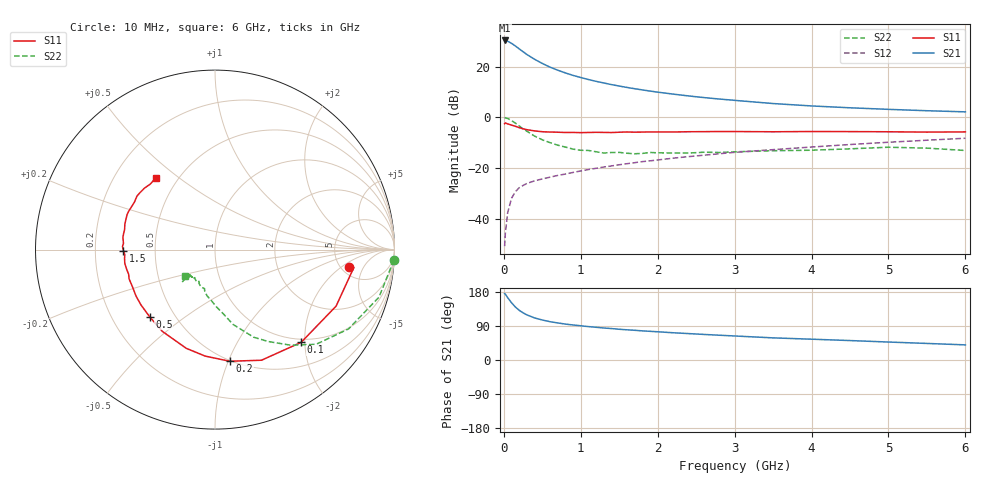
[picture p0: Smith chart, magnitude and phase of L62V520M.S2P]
!  INFINEON TECHNOLOGIES Small Signal Semiconductors
! BFR380L3 , Si-NPN RF-Transistor in TSLP-3-1
!  Vce=2.5 V,  Ic=20 mA
! Common Emitter S-Parameters:  07. March 2005
#  GHz  S  MA  R  50
! f  S11  S21  S12  S22
! GHz  Mag  Ang  Mag  Ang  Mag  Ang  Mag  Ang
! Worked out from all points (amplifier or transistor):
!   36 points, 10 MHz to 6 GHz, reference 50 ohm
!   highest |S21| = 30.3 dB at 10 MHz (marker M1)
!   |S21| within 3 dB of that: start of sweep to 185.8 MHz
!   unconditionally stable (mu >= 1): 1.909 GHz to 4.837 GHz
!   at 250 MHz: K = 0.37, MSG = 26.4 dB, |S12| = -26.8 dB
!   at 1.4 GHz: K = 0.95, MSG = 16.0 dB, |S12| = -19.1 dB
!   at 6 GHz: K = 0.97, MSG = 5.2 dB, |S12| = -8.2 dB
!   S11 on the Smith chart (normalised r, x): 10 MHz: 5.84, -2.59; 100 MHz: 0.94, -1.92; 200 MHz: 0.49, -1.01; 500 MHz: 0.36, -0.37; 1.5 GHz: 0.32, -0.00; 6 GHz: 0.38, +0.42
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0.01  0.7505 -7.4  32.83 175.0  0.0029 87.4  0.9974 -3.3
0.02  0.7797 -7.4  32.75 173.8  0.0053 84.4  0.981 -6.7
0.05  0.7446 -25.0  31.62 164.5  0.0133 81.4  0.9511 -16.2
0.1  0.7053 -47.1  28.82 151.1  0.0255 69.1  0.8655 -30.7
0.15  0.6686 -67.2  25.57 139.8  0.0344 62.0  0.772 -43.1
0.2  0.6274 -82.5  22.38 131.1  0.0411 58.7  0.6799 -51.6
0.25  0.5959 -95.3  19.7 124.5  0.0456 53.7  0.592 -59.9
0.3  0.5727 -106.3  17.35 119.0  0.0499 52.7  0.5335 -66.2
0.4  0.5419 -122.8  13.95 111.0  0.0563 50.6  0.4283 -76.5
0.5  0.522 -134.3  11.57 105.5  0.0613 50.9  0.3618 -82.5
0.6  0.5148 -143.3  9.787 101.1  0.0664 51.9  0.3182 -88.7
0.8  0.5044 -155.9  7.529 94.8  0.0765 54.3  0.2602 -100.0
0.9  0.5057 -161.3  6.72 92.4  0.0823 55.7  0.2372 -104.0
1.1  0.5046 -167.8  5.574 88.1  0.0939 57.8  0.2233 -110.0
1.5  0.5103 -179.4  4.15 81.1  0.1166 60.6  0.2045 -120.3
1.8  0.5139 174.3  3.483 76.9  0.1344 61.5  0.195 -125.8
2.2  0.516 167.4  2.878 71.9  0.1572 62.4  0.1992 -129.3
2.8  0.5272 158.2  2.303 65.4  0.1921 63.2  0.2037 -136.2
3.5  0.521 149.4  1.875 58.4  0.2316 61.9  0.2204 -135.7
4.5  0.5249 142.9  1.547 51.3  0.2921 61.0  0.2402 -135.6
5.5  0.5131 134.7  1.354 43.7  0.3552 57.7  0.248 -135.7
6  0.5182 129.3  1.286 39.9  0.3884 55.7  0.2228 -137.8
